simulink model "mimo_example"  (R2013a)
settings: Solver=ode45  StartTime=0.0  StopTime=10.0  RelTol=1e-3
libraries: simulink x4

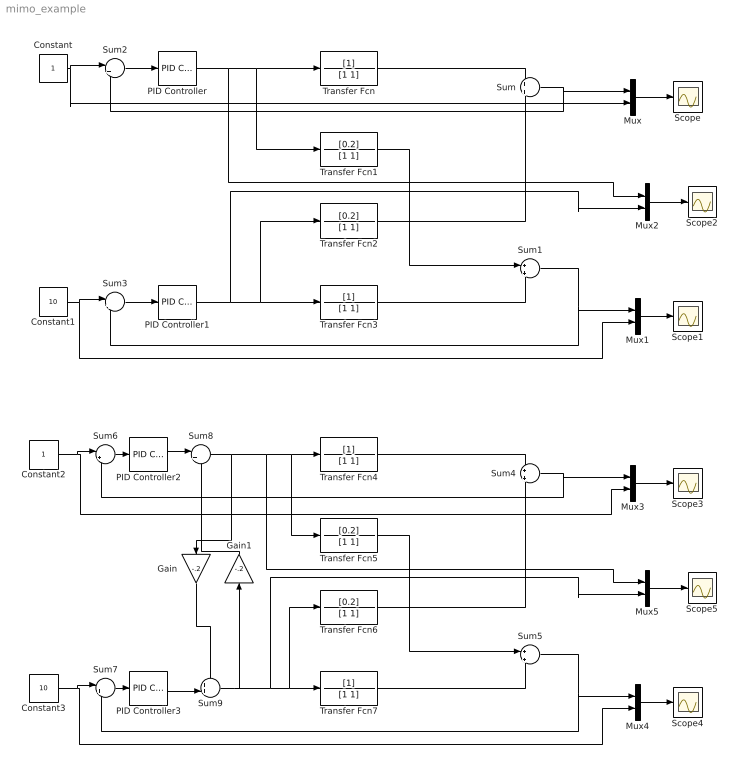
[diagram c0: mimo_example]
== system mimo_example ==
  Constant : Constant
  Constant1 : Constant  Value=10
  Constant2 : Constant
  Constant3 : Constant  Value=10
  Gain : Gain  Gain=-.2
  Gain1 : Gain  Gain=-.2
  Mux{,1..5} (6 alike) : Mux  Inputs=2
  PID Controller{,1..3} (4 alike) : simulink/Continuous/PID Controller  Controller=PID  TimeDomain=Continuous-time  SampleTime=1  IntegratorMethod=Forward Euler  FilterMethod=Forward Euler  Form=Parallel  P=1  I=1  D=0  N=100  InitialConditionSource=internal  InitialConditionForIntegrator=0  InitialConditionForFilter=0  ExternalReset=none  LimitOutput=off  UpperSaturationLimit=inf  LowerSaturationLimit=-inf  LinearizeAsGain=on  AntiWindupMode=none  Kb=1  TrackingMode=off  Kt=1  PParamMin=[]  PParamMax=[]  IParamMin=[]  IParamMax=[]  DParamMin=[]  DParamMax=[]  NParamMin=[]  NParamMax=[]  KbParamMin=[]  KbParamMax=[]  KtParamMin=[]  KtParamMax=[]  POutMin=[]  POutMax=[]  IOutMin=[]  IOutMax=[]  DOutMin=[]  DOutMax=[]  NOutMin=[]  NOutMax=[]  KbOutMin=[]  KbOutMax=[]  KtOutMin=[]  KtOutMax=[]  IntegratorOutMin=[]  IntegratorOutMax=[]  FilterOutMin=[]  FilterOutMax=[]  SumOutMin=[]  SumOutMax=[]  SumI1OutMin=[]  SumI1OutMax=[]  SumI2OutMin=[]  SumI2OutMax=[]  SumI3OutMin=[]  SumI3OutMax=[]  SumDOutMin=[]  SumDOutMax=[]  SaturationOutMin=[]  SaturationOutMax=[]  IntegratorContinuousStateAttributes=''  IntegratorStateMustResolveToSignalObject=off  IntegratorRTWStateStorageClass=Auto  FilterContinuousStateAttributes=''  FilterStateMustResolveToSignalObject=off  FilterRTWStateStorageClass=Auto
  Scope{,1..5} (6 alike) : Scope
  Sum{,1,4..5} (4 alike) : Sum  Inputs=+|+
  Sum{2..3,6..7} (4 alike) : Sum  Inputs=|+-
  Sum8 : Sum  Inputs=|++
  Sum9 : Sum  Inputs=++|
  Transfer Fcn{,3..4,7} (4 alike) : TransferFcn  Denominator=[1 1]
  Transfer Fcn{1..2,5..6} (4 alike) : TransferFcn  Numerator=[0.2]  Denominator=[1 1]
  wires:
  PID Controller1/1 -> Mux2/2, Transfer Fcn2/1, Transfer Fcn3/1
  PID Controller/1 -> Mux2/1, Transfer Fcn1/1, Transfer Fcn/1
  Sum/1 -> Sum2/2, Mux/1
  Transfer Fcn2/1 -> Sum/2
  Transfer Fcn/1 -> Sum/1
  Transfer Fcn1/1 -> Sum1/1
  Transfer Fcn3/1 -> Sum1/2
  Sum1/1 -> Mux1/1, Sum3/2
  Constant/1 -> Mux/2, Sum2/1
  Constant1/1 -> Mux1/2, Sum3/1
  Sum2/1 -> PID Controller/1
  Sum3/1 -> PID Controller1/1
  Mux/1 -> Scope/1
  Mux1/1 -> Scope1/1
  Mux2/1 -> Scope2/1
  Sum9/1 -> Gain1/1, Mux5/2, Transfer Fcn6/1, Transfer Fcn7/1
  Sum8/1 -> Gain/1, Mux5/1, Transfer Fcn5/1, Transfer Fcn4/1
  Sum4/1 -> Sum6/2, Mux3/1
  Transfer Fcn6/1 -> Sum4/2
  Transfer Fcn4/1 -> Sum4/1
  Transfer Fcn5/1 -> Sum5/1
  Transfer Fcn7/1 -> Sum5/2
  Sum5/1 -> Mux4/1, Sum7/2
  Constant2/1 -> Mux3/2, Sum6/1
  Constant3/1 -> Mux4/2, Sum7/1
  Sum6/1 -> PID Controller2/1
  Sum7/1 -> PID Controller3/1
  Mux3/1 -> Scope3/1
  Mux4/1 -> Scope4/1
  Mux5/1 -> Scope5/1
  PID Controller2/1 -> Sum8/1
  PID Controller3/1 -> Sum9/2
  Gain/1 -> Sum9/1
  Gain1/1 -> Sum8/2
